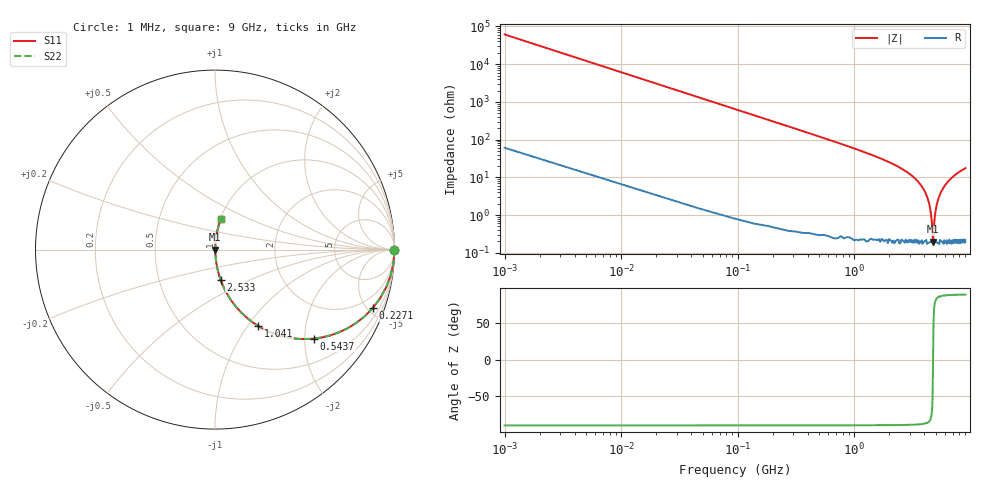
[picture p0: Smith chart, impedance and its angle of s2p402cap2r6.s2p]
! AVX Thin Film Operation		Date: December 2010
! Description: Accu-P® Series, Thin Film, SMD, RF Capacitor
! Part Number: 04021J2R6ABS
! 50 MHz  -  9 GHz
! Serial Measurements
# MHZ S MA R 50
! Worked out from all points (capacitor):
!   200 points, 1 MHz to 9 GHz, reference 50 ohm
!   read as one part in series: C = 2.6 pF near 46.22 MHz
!   lowest |Z| = 199 mohm at 4.749 GHz (marker M1)
!   series resonance near 4.751 GHz, so ESL is about 430 pH
!   S11 on the Smith chart (normalised r, x): 1 MHz: open; 227.1 MHz: 1.01, -5.38; 543.7 MHz: 1.01, -2.22; 1.041 GHz: 1.00, -1.12; 2.533 GHz: 1.00, -0.35; 9 GHz: 1.00, +0.35
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1  1 -0.1  0.001634 89.8  0.001634 89.8  1 -0.1
46.221  0.997 -4.3  0.075 85.6  0.075 85.6  0.997 -4.3
91.442  0.989 -8.5  0.148 81.4  0.148 81.4  0.989 -8.5
136.663  0.976 -12.6  0.218 77.3  0.218 77.3  0.976 -12.6
227.106  0.937 -20.4  0.348 69.5  0.348 69.5  0.937 -20.4
362.769  0.858 -30.8  0.512 59.1  0.512 59.1  0.858 -30.8
543.653  0.742 -41.9  0.668 47.9  0.668 47.9  0.742 -41.9
1041.085  0.488 -60.6  0.871 29.2  0.871 29.2  0.488 -60.6
1538.518  0.335 -70.1  0.94 19.6  0.94 19.6  0.335 -70.1
2533.382  0.17 -79.5  0.983 9.8  0.983 9.8  0.17 -79.5
3030.814  0.119 -82.2  0.991 6.8  0.991 6.8  0.119 -82.2
3980.457  0.046 -84.9  0.997 2.6  0.997 2.6  0.046 -84.9
4251.784  0.029 -84.4  0.998 1.6  0.998 1.6  0.029 -84.4
4523.111  0.013 -80.4  0.998 0.7  0.998 0.7  0.013 -80.4
4658.774  0.005408 -68.4  0.998 0.3  0.998 0.3  0.005408 -68.4
4749.216  0.001966 -2.7  0.998 0.0  0.998 0.0  0.001966 -2.7
4884.879  0.007415 74.2  0.998 -0.4  0.998 -0.4  0.007415 74.2
5065.764  0.017 82.3  0.998 -0.9  0.998 -0.9  0.017 82.3
5472.754  0.037 84.8  0.997 -2.1  0.997 -2.1  0.037 84.8
6015.407  0.061 84.7  0.996 -3.5  0.996 -3.5  0.061 84.7
7507.704  0.121 82.1  0.991 -6.9  0.991 -6.9  0.121 82.1
9000  0.173 79.4  0.983 -10.0  0.983 -10.0  0.173 79.4
